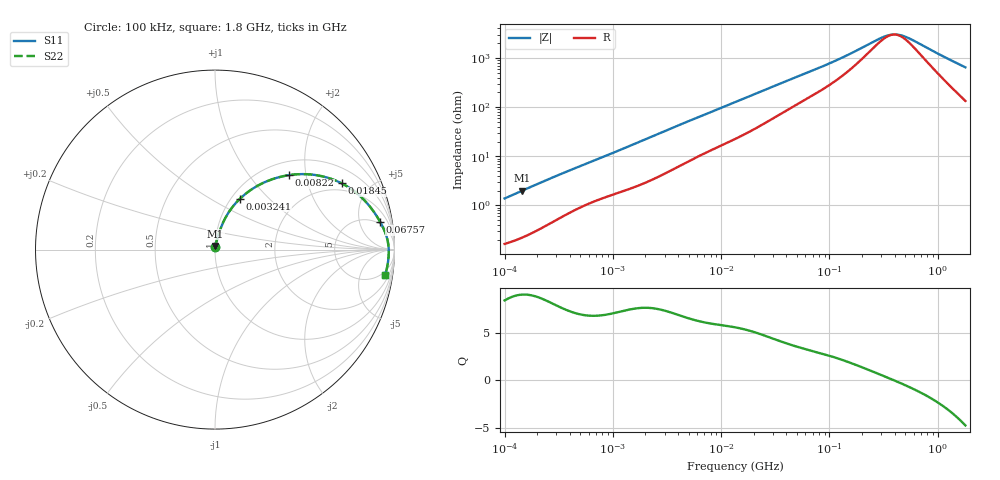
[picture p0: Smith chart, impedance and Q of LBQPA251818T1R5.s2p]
! LBQPA251818T1R5  S-PARAMETER MODEL  ( General Type )
! Model Generated by TAIYO YUDEN Corporation (http://www.ty-top.com)
! Version 1.0
! TAIYO YUDEN Control No. 191025NI43SB-FBB
! Copyright(c) 2019 TAIYO YUDEN CO.,LTD. All Rights Reserved.
! Product Description (link to TY-COMPAS)
! https://ds.yuden.co.jp/TYCOMPAS/or/detail?pn=LBQPA251818T1R5M&u=M
! Products Name : Inductors
! Characteristics :
!  Inductance : 1.5 uH , SRF(min) : 80 MHz , DC Resistance(max) : 0.143 Ohm
!  Rated Current : Saturation :950 mA , Temp Rise : 730 mA (20 degC)
!  Case Size : 2.5 x 1.8 / 0.098 x 0.071 [mm/inch] , Thickness : 1.8 / 0.071 [mm/inch]
!  (Conditions: Temperature = 25 degC , DC Bias Current/Voltage = 0A / 0V)
! External Node Assignments :
!  1  o---GGG---o  2
! GND o---------o GND
! Frequency Range : 0.1MHz  -  1800MHz  [ 402 STEP ]
# MHz S RI R 50
! Freq[MHz].  S11 Real  S11 Imag  S21 Real  S21 Imag  S12 Real  S12 Imag  S22 Real  S22 Imag
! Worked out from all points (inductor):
!   401 points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, 100 kHz to 1.8 GHz, reference 50 ohm
!   read as one part in series: L = 2.18 uH near 105 kHz
!   highest Q = 8.97 at 144.4 kHz (marker M1), where L = 2.17 uH
!   self-resonance near 393.6 MHz
!   S11 on the Smith chart (normalised r, x): 100 kHz: 1.00, +0.03; 3.241 MHz: 1.10, +0.69; 8.22 MHz: 1.27, +1.60; 18.45 MHz: 1.64, +3.32; 67.57 MHz: 4, +10; 1.8 GHz: 4, -13
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0.1  0.00183 0.0137  0.9982 -0.0137  0.9982 -0.0137  0.00183 0.0137
0.144402  0.00258 0.0196  0.9974 -0.0196  0.9974 -0.0196  0.00258 0.0196
0.516129  0.0133 0.0629  0.9867 -0.0629  0.9867 -0.0629  0.0133 0.0629
1.216451  0.0367 0.1311  0.9633 -0.1311  0.9633 -0.1311  0.0367 0.1311
1.844776  0.0633 0.1864  0.9367 -0.1864  0.9367 -0.1864  0.0633 0.1864
2.66389  0.1062 0.2481  0.8938 -0.2481  0.8938 -0.2481  0.1062 0.2481
3.240572  0.1396 0.2839  0.8604 -0.2839  0.8604 -0.2839  0.1396 0.2839
5.03627  0.2466 0.3607  0.7534 -0.3607  0.7534 -0.3607  0.2466 0.3607
8.220015  0.4116 0.4148  0.5884 -0.4148  0.5884 -0.4148  0.4116 0.4148
13.41641  0.5978 0.4084  0.4022 -0.4084  0.4022 -0.4084  0.5978 0.4084
18.44729  0.7063 0.369  0.2937 -0.369  0.2937 -0.369  0.7063 0.369
24.75089  0.7854 0.3179  0.2146 -0.3179  0.2146 -0.3179  0.7854 0.3179
33.20848  0.8429 0.2635  0.1571 -0.2635  0.1571 -0.2635  0.8429 0.2635
67.57036  0.9207 0.1534  0.0793 -0.1534  0.0793 -0.1534  0.9207 0.1534
69.24595  0.9224 0.1503  0.0776 -0.1503  0.0776 -0.1503  0.9224 0.1503
124.6553  0.9516 0.0859  0.0484 -0.0859  0.0484 -0.0859  0.9516 0.0859
286.6876  0.9665 0.0207  0.0335 -0.0207  0.0335 -0.0207  0.9665 0.0207
357.3983  0.9677 0.00624  0.0323 -0.00624  0.0323 -0.00624  0.9677 0.00624
424.248  0.9681 -0.00485  0.0319 0.00485  0.0319 0.00485  0.9681 -0.00485
516.0898  0.9681 -0.0178  0.0319 0.0178  0.0319 0.0178  0.9681 -0.0178
1186.925  0.9612 -0.0867  0.0388 0.0867  0.0388 0.0867  0.9612 -0.0867
1800  0.9488 -0.1388  0.0512 0.1388  0.0512 0.1388  0.9488 -0.1388
